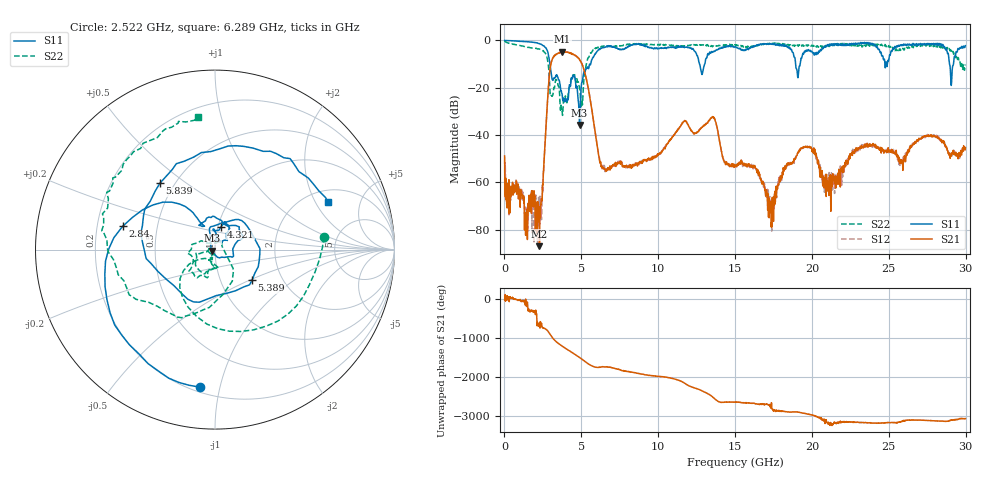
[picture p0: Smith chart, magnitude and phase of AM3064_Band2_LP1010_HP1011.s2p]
# Hz S DB R 50.0
!freq dBS11 angS11 dBS21 angS21 dBS12 angS12 dBS22 angS22
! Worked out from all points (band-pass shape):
!   1600 points, 10 MHz to 29.98 GHz, reference 50 ohm
!   highest |S21| = -4.80 dB at 3.759 GHz (marker M1); lowest = -86.9 dB at 2.278 GHz (marker M2)
!   |S21| within 3 dB of the highest: 3.121 GHz to 4.856 GHz (1.734 GHz wide, 43.5 % of centre)
!   lowest |S11| = -35.7 dB at 4.883 GHz (marker M3), VSWR 1.03, Z = 48.5 - j0.56 ohm
!   |S11| at or under -10 dB: 2.957 GHz to 5.61 GHz (2.654 GHz wide, 62 % of centre); 12.69 GHz to 13.03 GHz (338.8 MHz wide, 2.64 % of centre); 18.94 GHz to 19.23 GHz (295.2 MHz wide, 1.55 % of centre)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
!   |S22| runs from -31.7 to -0.3 dB; largest |S21 - S12| = 0.019
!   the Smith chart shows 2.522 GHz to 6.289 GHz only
!   S11 on the Smith chart (normalised r, x): 2.522 GHz: 0.23, -0.87; 2.84 GHz: 0.31, +0.11; 4.321 GHz: 1.03, +0.27; 5.389 GHz: 1.41, -0.52; 5.839 GHz: 0.42, +0.40; 6.289 GHz: 2.55, +2.55
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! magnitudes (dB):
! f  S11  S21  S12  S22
! 10 MHz  0.0  -48.8  -58.5  -0.3
! 2.278 GHz  -1.4  -86.9  -71.2  -3.6
! 2.522 GHz  -2.3  -57.2  -57.4  -4.3
! 2.84 GHz  -5.5  -21.5  -21.4  -9.8
! 3.759 GHz  -23.1  -4.8  -5.0  -30.5
! 4.321 GHz  -17.5  -5.4  -5.5  -16.7
! 4.883 GHz  -35.7  -8.1  -8.1  -20.4
! 5.015 GHz  -18.3  -9.7  -9.5  -25.8
! 5.389 GHz  -11.5  -18.3  -18.2  -8.3
! 5.839 GHz  -6.4  -36.0  -36.0  -3.6
! 6.289 GHz  -3.3  -53.4  -52.8  -2.6
! 10 GHz  -3.4  -48.1  -48.1  -1.9
! 13.54 GHz  -5.0  -32.5  -32.3  -2.6
! 15 GHz  -2.6  -52.7  -52.4  -1.9
! 16.34 GHz  -2.4  -54.0  -53.7  -2.4
! 17.37 GHz  -1.6  -76.9  -70.4  -1.2
! 19.99 GHz  -4.6  -45.8  -45.8  -2.0
! 21.08 GHz  -2.3  -61.8  -60.9  -2.1
! 25 GHz  -8.3  -47.0  -47.5  -2.2
! 28.28 GHz  -1.3  -41.4  -41.7  -3.2
! 29.08 GHz  -17.8  -48.0  -47.8  -5.0
! 29.98 GHz  -2.3  -45.3  -45.7  -10.2
